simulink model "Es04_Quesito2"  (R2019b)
settings: Solver=ode4  StartTime=0.0  StopTime=150  FixedStep=0.0001  RelTol=1e-3
undefined symbols (not defined in the file or in its folder): Tc1, Tc2, Tc3

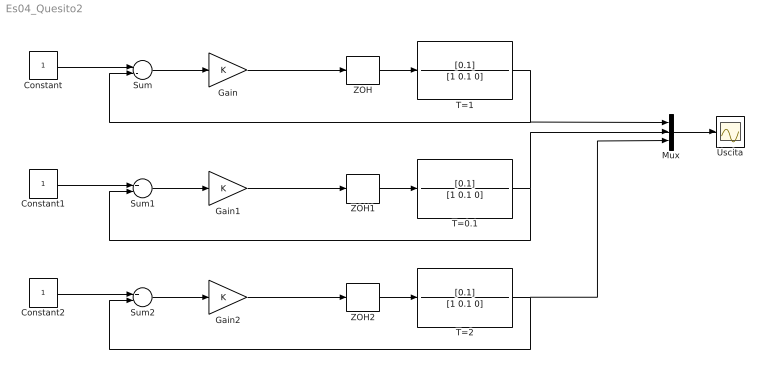
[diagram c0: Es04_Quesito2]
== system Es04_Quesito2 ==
  Constant : Constant
  Constant1 : Constant
  Constant2 : Constant
  Gain : Gain
  Gain1 : Gain
  Gain2 : Gain
  Mux : Mux  Inputs=3
  Sum : Sum  Inputs=+-
  Sum1 : Sum  Inputs=+-
  Sum2 : Sum  Inputs=+-
  T=0.1 : TransferFcn  Numerator=[0.1]  Denominator=[1 0.1 0]
  T=1 : TransferFcn  Numerator=[0.1]  Denominator=[1 0.1 0]
  T=2 : TransferFcn  Numerator=[0.1]  Denominator=[1 0.1 0]
  Uscita : Scope
  ZOH : ZeroOrderHold  SampleTime=Tc1
  ZOH1 : ZeroOrderHold  SampleTime=Tc2
  ZOH2 : ZeroOrderHold  SampleTime=Tc3
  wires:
  ZOH/1 -> T=1/1
  Sum/1 -> Gain/1
  T=1/1 -> Mux/1, Sum/2
  Constant/1 -> Sum/1
  Mux/1 -> Uscita/1
  Gain/1 -> ZOH/1
  T=0.1/1 -> Mux/2, Sum1/2
  Gain1/1 -> ZOH1/1
  Constant1/1 -> Sum1/1
  Sum1/1 -> Gain1/1
  ZOH1/1 -> T=0.1/1
  ZOH2/1 -> T=2/1
  Sum2/1 -> Gain2/1
  Constant2/1 -> Sum2/1
  Gain2/1 -> ZOH2/1
  T=2/1 -> Sum2/2, Mux/3
